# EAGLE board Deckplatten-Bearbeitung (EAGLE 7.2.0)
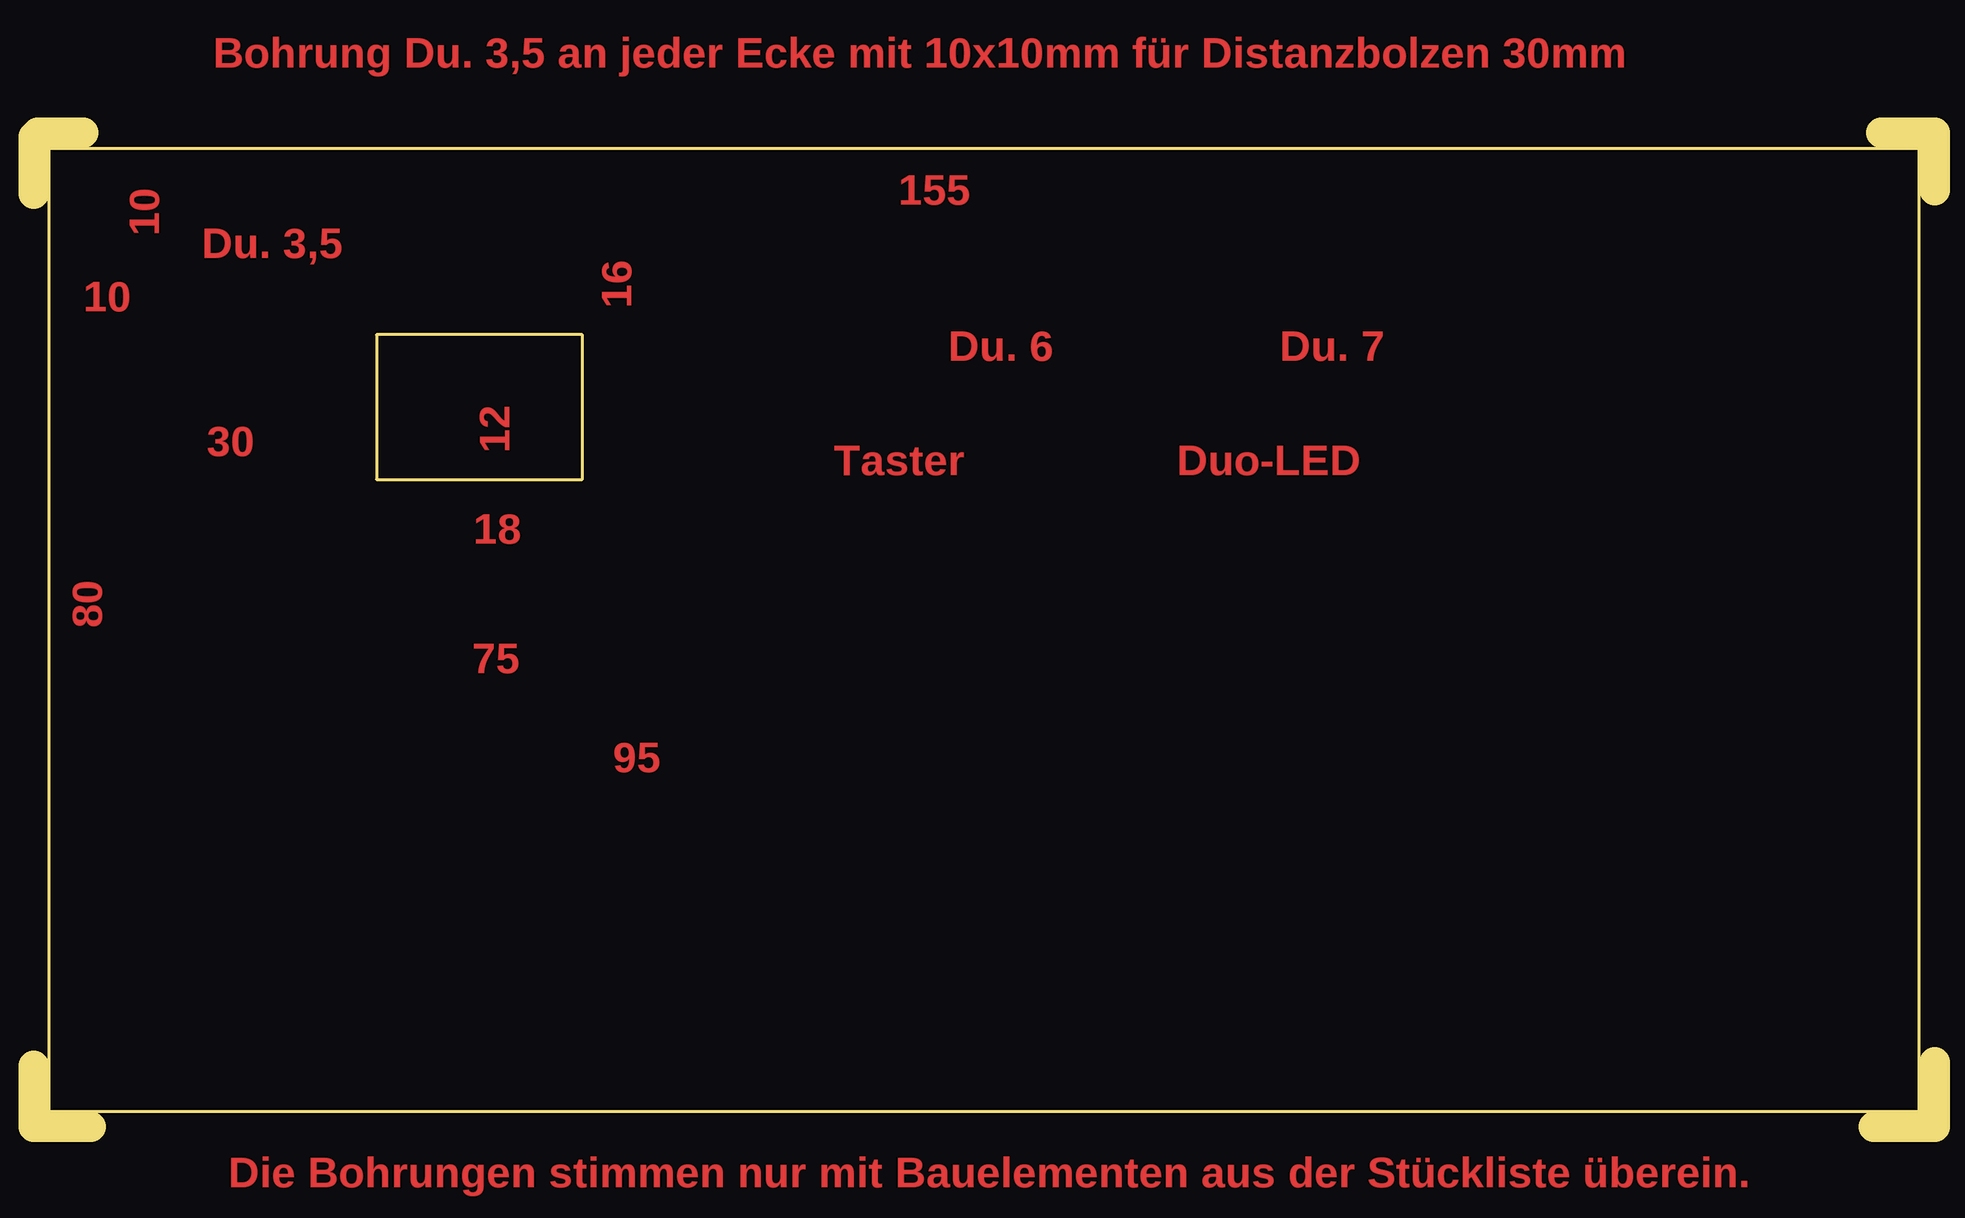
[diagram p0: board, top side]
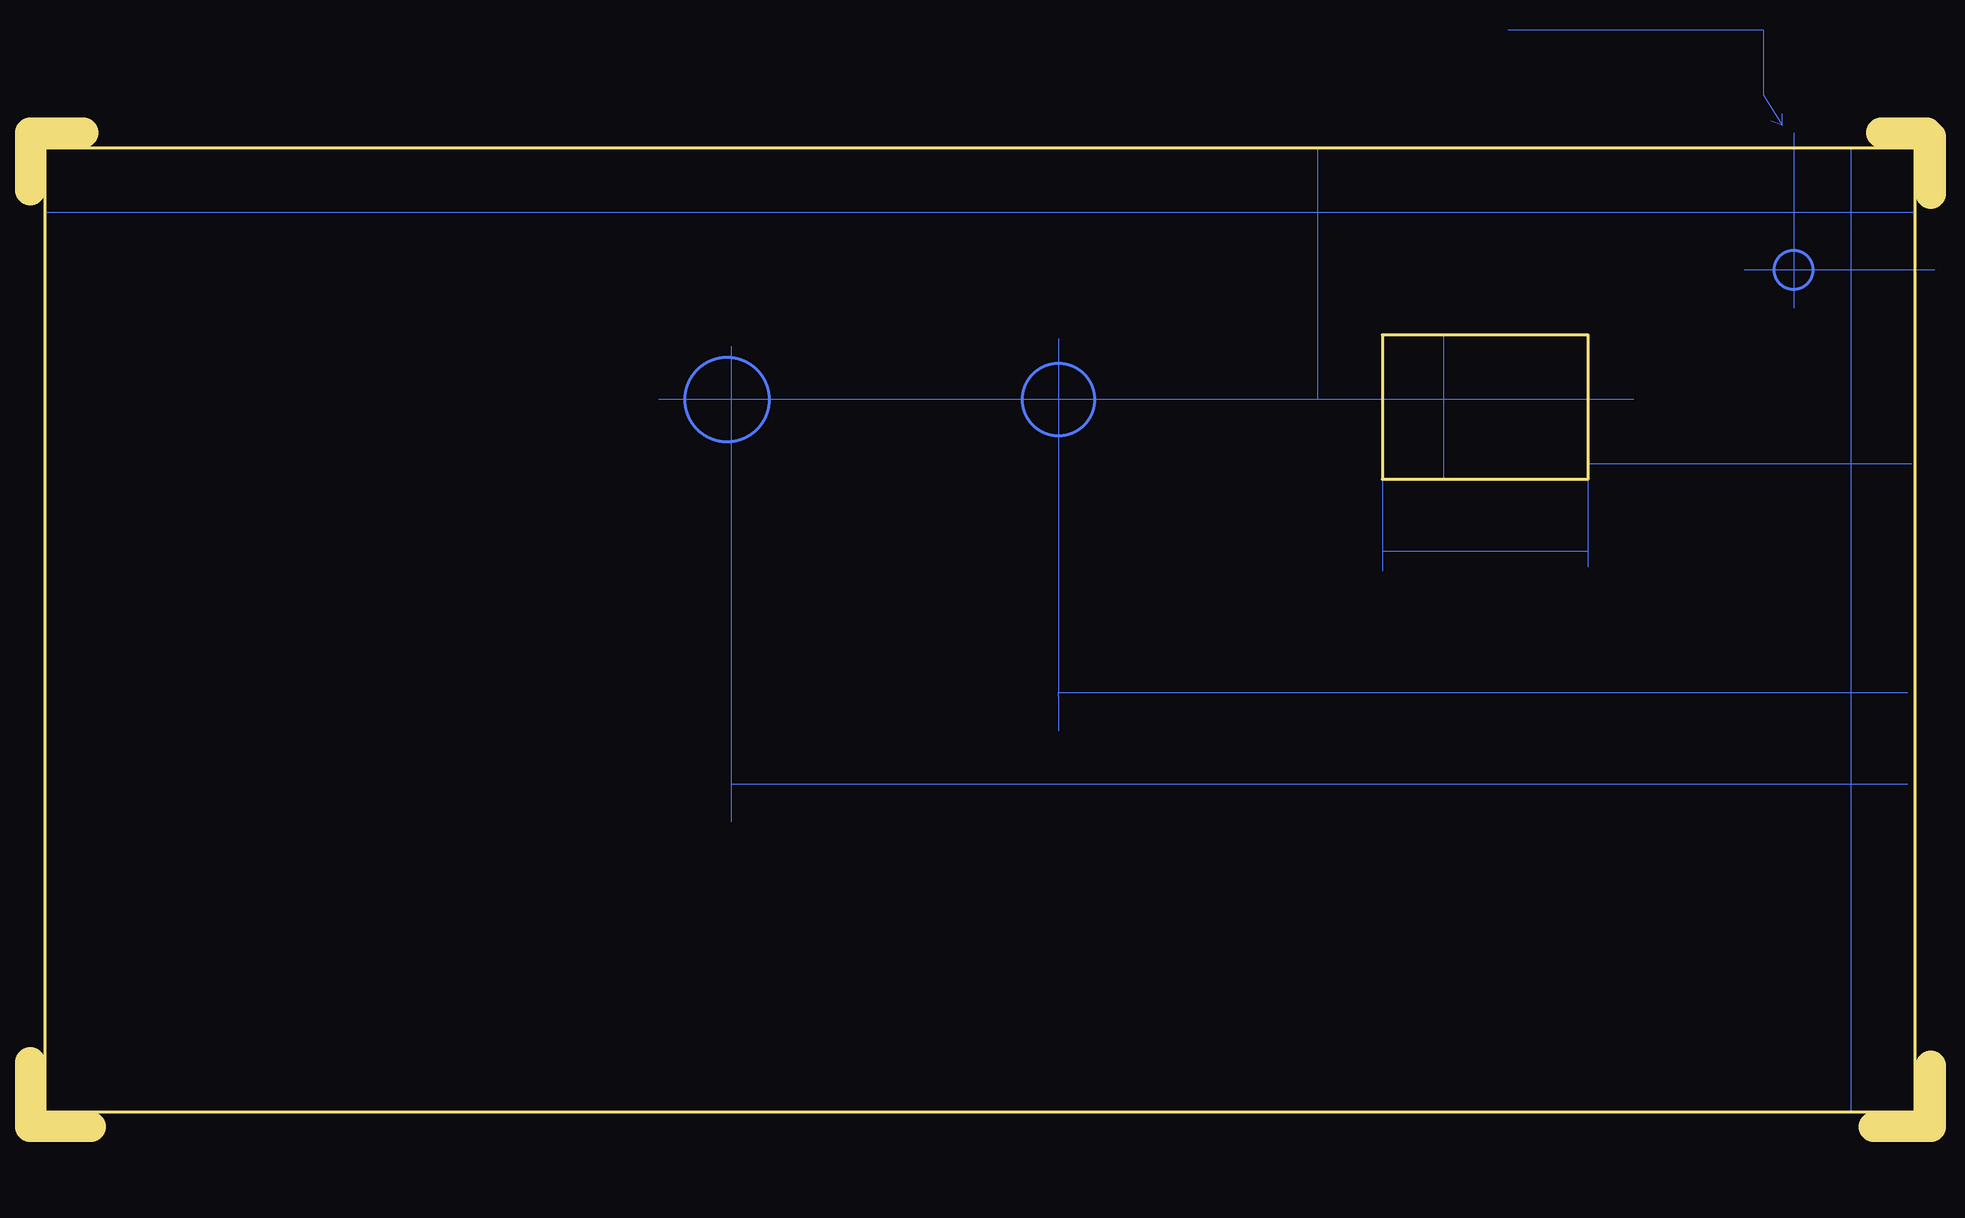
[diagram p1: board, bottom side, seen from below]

Size 158.43 x 82.87 mm. Coordinates in mm from the lower left corner, seen from the top.
Outline: 158.43,5.4 158.43,0.32
Outline: 158.43,0 153.35,0
Outline: 158.43,78.1 158.43,82.87 153.99,82.87
Outline: 0,5.08 0,0 4.76,0
Outline: 4.13,82.87 0.32,82.87
Outline: 0,77.79 0,82.55
Outline: 157.16,1.27 157.16,81.6 1.27,81.6 1.27,1.27 157.16,1.27
Outline: 45.72,66.04 45.72,53.98 28.57,53.98 28.57,66.04 45.72,66.04
Copper layers (1*16): Top 0.035mm / dielectric 1.5mm / Bottom 0.035mm
Design rules "default": minimum track width 10mil, minimum drill 24mil, track to track 8mil, track to pad 8mil, pad to pad 8mil, via to via 8mil, smd to smd 8mil, copper to edge 40mil, drill to drill 8mil, minimum pad ring 10mil, minimum via ring 8mil, stop-mask expansion 4mil, vias tented up to drill 0mil, thermal gap 10mil

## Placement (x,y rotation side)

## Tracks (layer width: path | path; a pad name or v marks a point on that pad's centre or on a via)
S$1
  Bottom 0: 28.57,54.29 28.57,47.94 | 28.57,47.94 28.57,46.67 | 45.72,53.98 45.72,47.94 | 45.72,47.94 45.72,46.36 | 28.57,47.94 45.72,47.94
S$2
  Bottom 0: 40.32,66.04 40.64,66.04 40.64,53.98
S$3
  Bottom 0: 1.59,55.25 28.57,55.25
S$4
  Bottom 0: 72.71,65.72 72.71,36.2 | 72.71,33.02 72.71,35.88 72.71,36.2 | 72.71,36.2 1.91,36.2
S$5
  Bottom 0: 24.77,60.64 51.12,60.64 | 51.12,60.64 106.05,60.64 | 51.12,81.6 51.12,60.64
S$6
  Bottom 0: 1.27,64.77 1.27,64.14
S$7
  Bottom 0: 1.27,76.2 157.16,76.2
S$8
  Bottom 0: 6.67,81.6 6.67,1.27
S$9
  Bottom 0: 100.01,65.09 100.01,28.57 | 100.01,28.57 100.01,25.4 | 100.01,28.57 1.91,28.57
S$22
  Bottom 0: 11.43,82.87 11.43,68.26
S$23
  Bottom 0: -0.32,71.44 15.56,71.44
S$24
  Bottom 0: 12.38,83.5 13.97,86.04 13.97,91.44 35.24,91.44 | 12.38,83.5 13.33,83.82 | 12.38,83.5 12.38,84.45
(copper drawn outside any net)
  shapes: Bottom circle x3

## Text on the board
Top: Alles so ungefähr. Aber NICHT masstabs-getreu ! | Die Abkürzung "Du." heißt Durchmesser | Bohrung Du. 3,5 an jeder Ecke mit 10x10mm für Distanzbolzen 30mm | 155 | 10 | Du. 3,5 | 10 | 16 | Du. 6 | Du. 7 | 30 | 12 | Taster | Duo-LED | 18 | 80 | 75 | 95 | Die Bohrungen stimmen nur mit Bauelementen aus der Stückliste überein.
